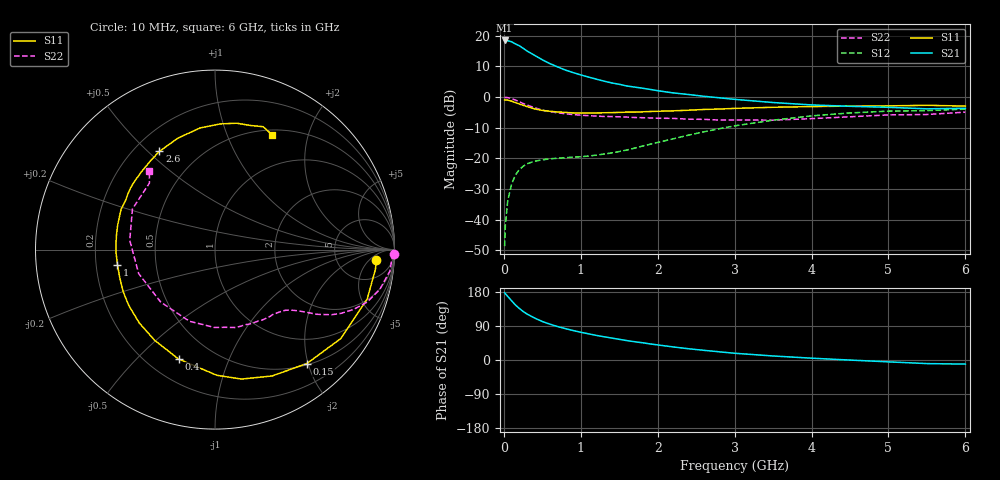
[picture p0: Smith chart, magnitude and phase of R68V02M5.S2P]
! SIEMENS Small Signal Semiconductors
! BFR193
! Si NPN RF Bipolar Junction Transistor in SOT23
! VCE = 8 V  IC = 2.5 mA
! Common Emitter S-Parameters:  May  1996
# GHz  S  MA  R  50
!  f  S11  S21  S12  S22
! GHz  MAG  ANG  MAG  ANG  MAG  ANG  MAG  ANG
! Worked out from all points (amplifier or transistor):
!   36 points, 10 MHz to 6 GHz, reference 50 ohm
!   highest |S21| = 18.5 dB at 10 MHz (marker M1)
!   |S21| within 3 dB of that: start of sweep to 276.1 MHz
!   unconditionally stable (mu >= 1): 1.116 GHz to 2.034 GHz
!   at 250 MHz: K = 0.27, MSG = 19.3 dB, |S12| = -22.6 dB
!   at 1.4 GHz: K = 1.10, MAG = 9.5 dB, |S12| = -18.2 dB
!   at 6 GHz: K = 0.98, MSG = 0.1 dB, |S12| = -3.9 dB
!   S11 on the Smith chart (normalised r, x): 10 MHz: 14, -9; 150 MHz: 0.52, -1.98; 400 MHz: 0.32, -0.67; 1 GHz: 0.29, -0.07; 2.6 GHz: 0.30, +0.54; 6 GHz: 0.56, +1.47
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0.01  0.9012 -3.8  8.405 177.8  0.0037 86.3  0.9963 -1.4
0.02  0.9004 -7.1  8.268 175.0  0.0081 84.3  0.9876 -2.8
0.05  0.8916 -18.0  8.324 167.9  0.0201 80.1  0.9816 -7.0
0.1  0.8583 -35.3  8.021 156.6  0.038 71.4  0.9445 -13.6
0.15  0.8155 -51.1  7.38 145.4  0.0534 63.9  0.8971 -19.0
0.2  0.7725 -65.7  6.908 136.3  0.0655 57.1  0.8418 -23.3
0.25  0.7363 -78.4  6.271 128.2  0.0742 51.5  0.7873 -26.8
0.3  0.7006 -89.1  5.671 121.5  0.0816 47.9  0.7441 -29.2
0.4  0.6427 -108.4  4.808 110.7  0.0902 41.9  0.6707 -32.5
0.5  0.607 -123.6  4.069 101.6  0.0946 38.9  0.6135 -34.6
0.6  0.5874 -135.9  3.518 94.5  0.0986 37.5  0.5784 -36.2
0.7  0.5728 -146.8  3.107 88.2  0.1006 37.1  0.555 -37.6
0.8  0.563 -155.4  2.765 82.8  0.1026 37.7  0.5354 -39.0
1  0.5499 -171.1  2.303 73.2  0.1065 41.4  0.5071 -42.4
1.1  0.5514 -178.1  2.126 69.1  0.1093 43.7  0.4981 -44.5
1.6  0.5696 156.6  1.519 51.2  0.1372 56.2  0.4724 -56.2
2.2  0.5973 133.0  1.173 34.5  0.2085 62.6  0.4501 -74.7
2.6  0.6288 119.5  1.032 25.6  0.2714 60.6  0.4339 -90.6
3.5  0.6831 96.9  0.816 10.6  0.4206 46.8  0.4208 -135.9
4.5  0.7144 80.3  0.708 -0.2  0.5523 27.0  0.4777 173.8
5.5  0.7353 68.6  0.644 -9.5  0.6023 7.8  0.5204 134.6
6  0.7138 63.4  0.658 -10.8  0.6365 2.6  0.5689 130.0
